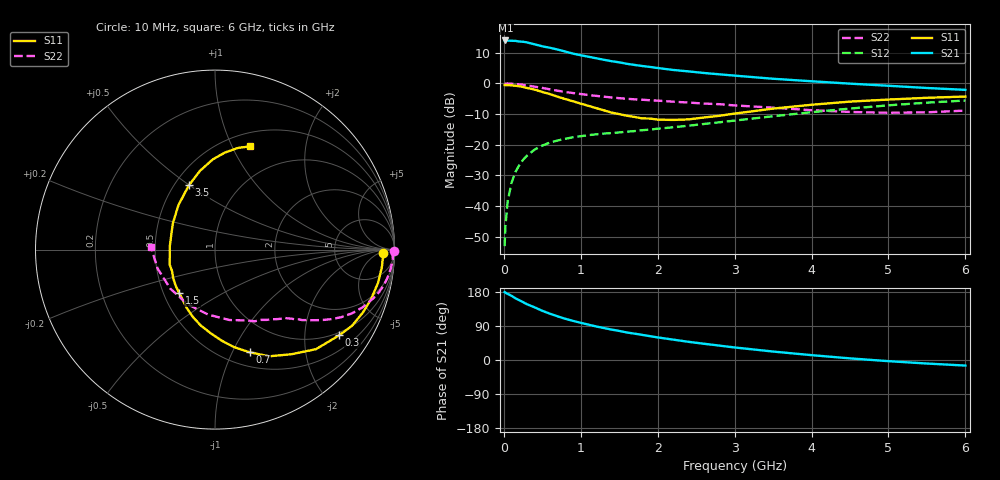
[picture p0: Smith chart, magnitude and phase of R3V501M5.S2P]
! SIEMENS Small Signal Semiconductors
! BFR181
! Si NPN RF Bipolar Junction Transistor in SOT23
! VCE = 0.5 V  IC = 1.5 mA
! Common Emitter S-Parameters:  May  1996
# GHz  S  MA  R  50
!  f  S11  S21  S12  S22
! GHz  MAG  ANG  MAG  ANG  MAG  ANG  MAG  ANG
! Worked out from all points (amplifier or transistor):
!   36 points, 10 MHz to 6 GHz, reference 50 ohm
!   highest |S21| = 14.0 dB at 20 MHz (marker M1)
!   |S21| within 3 dB of that: start of sweep to 704.7 MHz
!   unconditionally stable (mu >= 1): 1.548 GHz to 4.258 GHz
!   at 250 MHz: K = 0.21, MSG = 19.3 dB, |S12| = -25.0 dB
!   at 1.4 GHz: K = 0.94, MSG = 11.7 dB, |S12| = -16.2 dB
!   at 6 GHz: K = 0.96, MSG = 1.7 dB, |S12| = -5.6 dB
!   S11 on the Smith chart (normalised r, x): 10 MHz: 28, -8; 300 MHz: 0.91, -2.96; 700 MHz: 0.65, -1.17; 1.5 GHz: 0.60, -0.32; 3.5 GHz: 0.59, +0.50; 6 GHz: 0.65, +1.18
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0.01  0.9369 -1.1  4.961 179.3  0.0022 91.3  0.9953 -0.6
0.02  0.9367 -2.5  5.005 177.6  0.0046 81.5  0.9892 -1.2
0.05  0.9349 -5.9  4.981 174.6  0.0119 85.5  0.9921 -3.1
0.1  0.9271 -11.5  4.944 169.4  0.0238 83.1  0.9851 -6.0
0.15  0.9122 -17.6  4.927 162.9  0.0356 78.7  0.9746 -9.1
0.25  0.8735 -29.1  4.769 152.6  0.0564 71.8  0.9446 -14.5
0.3  0.8407 -34.6  4.654 147.3  0.0658 69.3  0.9239 -17.0
0.4  0.7901 -44.6  4.332 138.9  0.0829 63.4  0.8825 -21.4
0.5  0.7223 -53.8  4.018 129.8  0.0964 58.9  0.8414 -25.0
0.6  0.6665 -63.1  3.803 122.1  0.108 54.6  0.7972 -28.2
0.7  0.6042 -71.3  3.556 115.1  0.1168 51.8  0.7563 -30.8
0.9  0.5093 -85.7  3.05 103.2  0.1318 47.3  0.694 -34.5
1.1  0.429 -100.9  2.716 93.3  0.1425 44.5  0.645 -37.5
1.3  0.3627 -115.5  2.423 84.4  0.1513 42.9  0.6052 -39.9
1.5  0.3143 -129.4  2.201 76.7  0.1579 42.6  0.5724 -42.2
1.9  0.266 -161.7  1.85 62.9  0.1758 43.0  0.5293 -46.8
2.2  0.2525 175.9  1.653 53.8  0.1916 43.9  0.5013 -50.8
2.8  0.2948 138.1  1.403 38.0  0.2311 44.6  0.4568 -61.0
3.5  0.3864 112.2  1.187 22.3  0.2902 42.7  0.4006 -78.4
4.5  0.5029 91.4  0.988 4.3  0.3874 34.9  0.3409 -116.7
5.5  0.5805 77.3  0.839 -9.3  0.4836 23.1  0.3366 -161.7
6  0.6082 71.1  0.782 -14.7  0.524 16.2  0.3588 177.3
